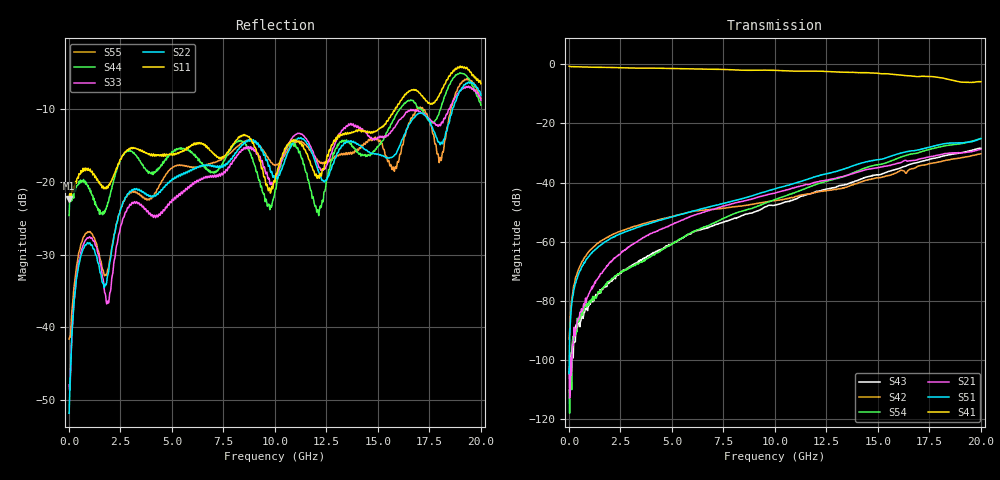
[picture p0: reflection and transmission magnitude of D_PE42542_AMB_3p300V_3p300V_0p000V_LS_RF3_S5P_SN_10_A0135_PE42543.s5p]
! Device ID: PE42542
! Device ID: PE42542
! File Path: z:\PE42542\PE42543_20140723_inv\AMB\3p300\LS_RF3\PE42542_AMB_3p300V_3p300V_0p000V_LS_RF3_S5P_SN_10_A0135_PE42543.s5p
! Serial: 10
! Lot: A0135_PE42543
! Temp: AMB
! VDD: 3.300
! VSS: 0.000
! Control_Hi: 3.300
! Control_Lo: 0.000
! Logic State: LS_RF3
! Port 1: RFC
! Port 2: RF1
! Port 3: RF2
! Port 5: RF3
! Port 6: RF4
! ThroughPath:1-5
! IDD: -0.000136002403
! ISS: 2.80847847e-009
#  Hz  S  RI  R  50
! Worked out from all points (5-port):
!   801 points, 10 MHz to 20 GHz, reference 50 ohm
!   strongest paths, dB at 10 MHz, 5.008 GHz, 10.01 GHz, 15 GHz, 20 GHz:
!     S41: -0.6, -1.4, -2.0, -3.1, -5.9
!     S51: -104.6, -51.6, -42.1, -32.3, -25.1
!     S21: -102.5, -54.3, -43.5, -35.0, -28.7
!     S54: -110.2, -60.9, -45.8, -34.0, -25.1
!     S42: -93.0, -51.5, -46.0, -38.4, -30.3
!     S43: -104.1, -60.8, -47.6, -37.5, -28.4
!   lowest |S11| = -22.3 dB at 10 MHz (marker M1), VSWR 1.17, Z = 57.9 - j2.4 ohm
!   |S11| at or under -10 dB: start of sweep to 15.84 GHz
